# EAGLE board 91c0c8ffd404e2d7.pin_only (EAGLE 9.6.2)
REV: A

Size 63.5 x 55.88 mm. Coordinates in mm from the lower left corner, seen from the top.
Outline: 2.54,55.88 60.96,55.88 arc-90 63.5,53.34 63.5,2.54 arc-90 60.96,0 arc-90 58.42,2.54 arc90 56.64,4.32 6.86,4.32 arc90 5.08,2.54 arc-90 2.54,0 arc-90 0,2.54 0,53.34 arc-90 2.54,55.88
Copper layers (1*16): Top 0.035mm / dielectric 1.5mm / Bottom 0.035mm
Design rules "adafruit 7-7": minimum track width 6mil, minimum drill 15.5mil, track to track 8mil, track to pad 7mil, pad to pad 7mil, via to via 7mil, smd to smd 7mil, copper to edge 10mil, drill to drill 8mil, minimum pad ring 10mil, minimum via ring 8mil, stop-mask expansion 2mil, vias tented up to drill 20mil, thermal gap 10mil

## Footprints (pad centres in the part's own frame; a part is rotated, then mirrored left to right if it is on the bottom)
0603-NO = smd 1.075 x 1: 1 -0.85,0; 2 0.85,0
0805_10MGAP = smd 1.2 x 1.5: 1 -1.05,0; 2 1.05,0
0805-NO = smd 1.24 x 1.5: 1 -0.95,0; 2 0.95,0
_0805 = smd 1.2 x 1.3: 1 -1.016,0; 2 1.016,0
FIDUCIAL_1MM = smd 1 x 1: 1 0,0
SHARP_2.7IN = smd 0.25 x 1.4: P$1 -2.25,2.9; P$2 -1.75,2.9; P$3 -1.25,2.9; P$4 -0.75,2.9; P$5 -0.25,2.9; P$6 0.25,2.9; P$7 0.75,2.9; P$8 1.25,2.9; P$9 1.75,2.9; P$10 2.25,2.9 | smd 1.6 x 2.2: SUPPORT1 -4.9,-0.25; SUPPORT2 4.9,-0.25
SOT23-6 = smd 0.55 x 1.2: 1 -0.95,-1.3; 2 0,-1.3; 3 0.95,-1.3; 4 0.95,1.3; 5 0,1.3; 6 -0.95,1.3
1X09_ROUND_70 = drill 1 pad 1.778: 1 -10.16,0; 2 -7.62,0; 3 -5.08,0; 4 -2.54,0; 5 0,0; 6 2.54,0; 7 5.08,0; 8 7.62,0; 9 10.16,0
SOIC16 = smd 0.6 x 2.2: 1 -4.445,-2.6; 2 -3.175,-2.6; 3 -1.905,-2.6; 4 -0.635,-2.6; 5 0.635,-2.6; 6 1.905,-2.6; 7 3.175,-2.6; 8 4.445,-2.6; 9 4.445,2.6; 10 3.175,2.6; 11 1.905,2.6; 12 0.635,2.6; 13 -0.635,2.6; 14 -1.905,2.6; 15 -3.175,2.6; 16 -4.445,2.6
SOT23-5 = smd 0.55 x 1.2: 1 -0.95,-1.3; 2 0,-1.3; 3 0.95,-1.3; 4 0.95,1.3; 5 -0.95,1.3
MOUNTINGHOLE_2.5_PLATED_THICK = drill 2.5 pad 4: P$1 0,0
MOUNTINGHOLE_2.5_PLATED = drill 2.5 pad 3.2: P$1 0,0

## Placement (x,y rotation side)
C1  0.1µF  [0603-NO]  30.2,21.34 90 top
C2  1µF  [0805_10MGAP]  33.66,18.19 0 top
C3  1µF  [0805-NO]  33.88,21.34 90 top
C4  10µF  [0805-NO]  40.99,40.83 180 top
C5  10µF  [0805-NO]  40.91,33.67 180 top
C6  10uF  [0805-NO]  45.47,33.66 0 top
C7  10uF  [0805-NO]  48.51,34.67 270 top
C8  1uF  [0805-NO]  45.72,40.89 180 top
FB1  FERRITE  [_0805]  31.97,21.34 270 top
FB2  FERRITE  [_0805]  35.91,21.34 270 top
FID1  FIDUCIAL_1MM  [FIDUCIAL_1MM]  2.94,47.68 180 top
FID2  FIDUCIAL_1MM  [FIDUCIAL_1MM]  61.12,9.47 180 top
FID3  FIDUCIAL_1MM  [FIDUCIAL_1MM]  61.09,48.77 180 top
IC1  LS013B4DN04  [SHARP_2.7IN]  31.75,12.19 0 top
IC2  AP3602  [SOT23-6]  45.72,37.21 0 top
JP1  [1X09_ROUND_70]  31.75,53.34 180 top
R1  10K  [0603-NO]  29.69,32.26 90 top
R2  10K  [0603-NO]  27.21,32.26 270 top
R3  10K  [0603-NO]  33.43,32.38 90 top
U1  74HC4050D  [SOIC16]  31.59,38.35 180 top
U2  AP2112K-3.3  [SOT23-5]  40.95,37.18 180 top
U$21  MOUNTINGHOLE2.5_THICK  [MOUNTINGHOLE_2.5_PLATED_THICK]  60.96,2.54 90 top
U$22  MOUNTINGHOLE2.5_THICK  [MOUNTINGHOLE_2.5_PLATED_THICK]  2.54,2.54 270 top
U$27  MOUNTINGHOLE2.5  [MOUNTINGHOLE_2.5_PLATED]  60.96,53.34 270 top
U$28  MOUNTINGHOLE2.5  [MOUNTINGHOLE_2.5_PLATED]  2.54,53.34 90 top
U$29  [PCBFEAT-REV-040]  32,27.05 0 top
U$32  [ADAFRUIT_TEXT_20MM]  2.29,29.59 0 top

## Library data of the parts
C1-C3 C6-C8 FB1 FB2 IC2 JP1 R1 R2 U1 U$29 U$32 = microbuilder
C4 C5 R3 = microbuilder; CHECKED: KTOWN; COMPANY: ADAFRUIT INDUSTRIES; DRAWN: KTOWN; REV: A
FID1 FID2 U$21 U$22 = microbuilder; BOM: EXCLUDE
FID3 U$27 U$28 = microbuilder; BOM: EXCLUDE; CHECKED: KTOWN; COMPANY: ADAFRUIT INDUSTRIES; DRAWN: KTOWN; REV: A
IC1 = adafruit_display
U2 = adafruit_power

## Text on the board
tPlace: CS | DISP | MOSI | SCLK | GND | 3V3 | EXTIN | EXTMD | VIN (3.3-5V) | 3 or 5V logic / CS is active high! | 2.7" 400x240 / SHARP Memory Display
bPlace: DISP | CS | CLK | 3v3 | EIN | EMD | DI | GND | VIN | Adafruit Sharp Memory Display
